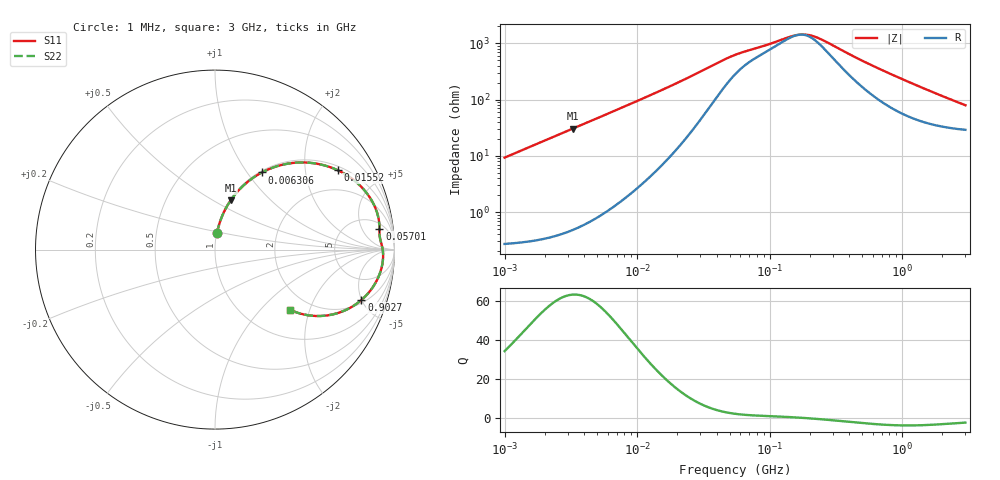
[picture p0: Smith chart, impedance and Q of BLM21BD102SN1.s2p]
! BLM21BD102SN1
# Hz S RI R 50
!Freq.(Hz) S11(Real) S11(Imag) S21(Real) S21(Imag) S12(Real) S12(Imag) S22(Real) S22(Imag)
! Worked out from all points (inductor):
!   401 points, 1 MHz to 3 GHz, reference 50 ohm
!   read as one part in series: L = 1.48 uH near 1.041 MHz
!   highest Q = 63.3 at 3.257 MHz (marker M1), where L = 1.48 uH
!   self-resonance near 167.5 MHz
!   S11 on the Smith chart (normalised r, x): 1 MHz: 1.01, +0.19; 6.306 MHz: 1.02, +1.18; 15.52 MHz: 1.14, +2.99; 57.01 MHz: 7, +11; 902.7 MHz: 2.27, -4.99; 3 GHz: 1.58, -1.48
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1000000  0.0112 0.0916  0.9888 -0.0916  0.9888 -0.0916  0.0112 0.0916
1822989  0.0308 0.1637  0.9692 -0.1637  0.9692 -0.1637  0.0308 0.1637
3257432  0.0877 0.2751  0.9123 -0.2751  0.9123 -0.2751  0.0877 0.2751
3823119  0.1163 0.3127  0.8837 -0.3127  0.8837 -0.3127  0.1163 0.3127
6305767  0.2618 0.4301  0.7382 -0.4301  0.7382 -0.4301  0.2618 0.4301
9794439  0.4613 0.485  0.5387 -0.485  0.5387 -0.485  0.4613 0.485
1.461624e7  0.6567 0.4537  0.3433 -0.4537  0.3433 -0.4537  0.6567 0.4537
1.55208e7  0.6832 0.4425  0.3168 -0.4425  0.3168 -0.4425  0.6832 0.4425
2.095589e7  0.7951 0.3688  0.2049 -0.3688  0.2049 -0.3688  0.7951 0.3688
2.773354e7  0.8646 0.2873  0.1354 -0.2873  0.1354 -0.2873  0.8646 0.2873
3.74453e7  0.9037 0.2036  0.0963 -0.2036  0.0963 -0.2036  0.9037 0.2036
5.477226e7  0.9162 0.1225  0.0838 -0.1225  0.0838 -0.1225  0.9162 0.1225
5.700937e7  0.9163 0.1161  0.0837 -0.1161  0.0837 -0.1161  0.9163 0.1161
1.520175e8  0.9327 0.011  0.0673 -0.011  0.0673 -0.011  0.9327 0.011
1.784169e8  0.9354 -0.00743  0.0646 0.00743  0.0646 0.00743  0.9354 -0.00743
2.094008e8  0.9367 -0.0272  0.0633 0.0272  0.0633 0.0272  0.9367 -0.0272
2.558035e8  0.9359 -0.0538  0.0641 0.0538  0.0641 0.0538  0.9359 -0.0538
4.480278e8  0.9149 -0.1422  0.0851 0.1422  0.0851 0.1422  0.9149 -0.1422
8.005644e8  0.8415 -0.2563  0.1585 0.2563  0.1585 0.2563  0.8415 -0.2563
9.0272e8  0.8161 -0.2805  0.1839 0.2805  0.1839 0.2805  0.8161 -0.2805
1.67892e9  0.623 -0.3669  0.377 0.3669  0.377 0.3669  0.623 -0.3669
3e9  0.4166 -0.3344  0.5834 0.3344  0.5834 0.3344  0.4166 -0.3344
